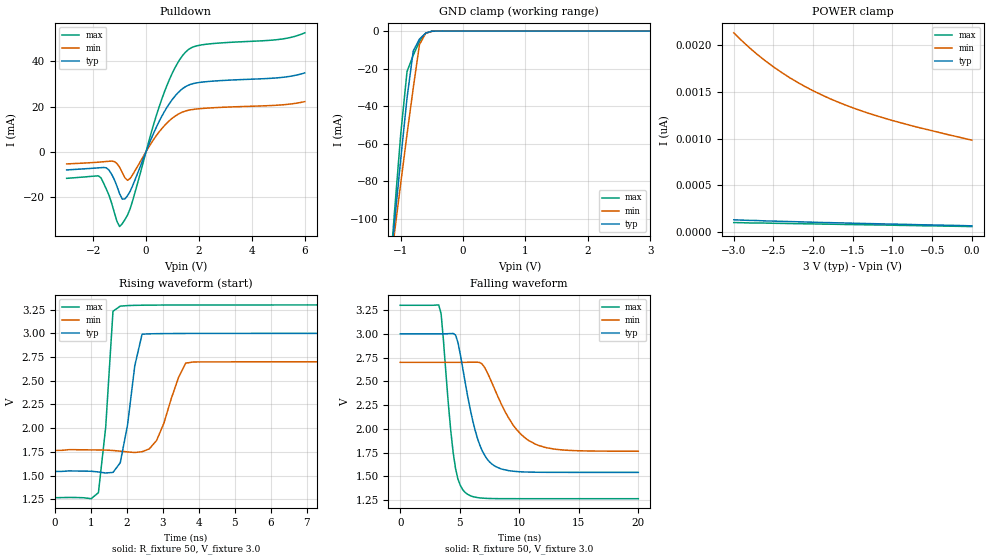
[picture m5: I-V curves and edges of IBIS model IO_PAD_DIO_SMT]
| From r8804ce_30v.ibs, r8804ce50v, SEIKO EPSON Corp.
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[Model]   IO_PAD_DIO_SMT
Model_type I/O_open_drain
Enable Active-High
Polarity Non-Inverting
Vinh=2.64
Vinl=0.54
Vref=3.3
Vmeas=1.50
Rref=5000
C_comp   2.5p   2.0p   3.0p
[Temperature Range] 25   105   -40
[Voltage Range]   3.0   2.7   3.3
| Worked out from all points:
|   slope of the pulldown table from 0 to 0.45 V, typ, clamps not added: 36.6 ohm
|   GND clamp passes 1 mA (typ) near -0.59 V on its own axis
|   falling waveform, R_fixture 50, V_fixture 3.0: 20-80 % time 1.52ns typ, 2.47ns min, 886ps max; typ from 3 V to 1.54 V
|   rising waveform, R_fixture 50, V_fixture 3.0: 20-80 % time 333ps typ, 498ps min, 245ps max; typ from 1.54 V to 3 V
[Pulldown]
-3V       -8.089mA   -5.43mA    -11.82mA
-1.7V     -7.088mA   -4.564mA   -11.64mA
-1.4V     -8.196mA   -4.255mA   -19.3mA
-1V       -18.62mA   -6.885mA   -33.2mA
-800mV    -20.97mA   -11.57mA   -30.13mA
-600mV    -17.54mA   -11.87mA   -25.25mA
600mV     15.77mA    10.27mA    23.45mA
1.1V      24.7mA     15.77mA    37.31mA
1.5V      28.87mA    18.05mA    44.2mA
2.1V      30.79mA    19.12mA    47.31mA
5V        32.75mA    20.62mA    49.7mA
6V        34.91mA    22.17mA    52.66mA
[GND Clamp]
-3V       -764.1mA   -630.2mA   -940.2mA
-1.2V     -136mA     -134.3mA   -139.6mA
-1.1V     -101.9mA   -107.4mA   -96.17mA
-1V       -68.05mA   -80.96mA   -54.69mA
-900mV    -35.72mA   -55.09mA   -21.63mA
-800mV    -10.59mA   -30.38mA   -12.89mA
-700mV    -4.3mA     -7.21mA    -5.615mA
-600mV    -1.094mA   -1.181mA   -1.208mA
-500mV    -109.6uA   -173.5uA   -67.33uA
-400mV    -6.015uA   -18.81uA   -1.378uA
3V        67.42pA    1.041nA    53.55pA
[POWER Clamp]
-3V       132.1pA    2.129nA    102.5pA
-2.8V     125.7pA    1.968nA    98.45pA
-2.7V     124.1pA    1.896nA    98.23pA
-2.5V     118.5pA    1.765nA    95.04pA
-2.3V     113.1pA    1.652nA    92.31pA
-2.2V     111.3pA    1.602nA    90.27pA
-2V       106.2pA    1.51nA     88.33pA
-1.8V     102pA      1.43nA     85.27pA
-1.4V     93.68pA    1.298nA    79.69pA
-1V       86.74pA    1.192nA    74.58pA
-700mV    80.26pA    1.124nA    70.03pA
0V        67.42pA    982.3pA    59.57pA
[Falling Waveform]
R_fixture=50
V_fixture=3.0
V_fixture_min=2.7
V_fixture_max=3.3
0s        3V         2.7V       3.3V
3.232ns   3V         2.7V       3.304V
3.434ns   3V         2.7V       3.212V
4.444ns   3.003V     2.7V       1.754V
5.455ns   2.49V      2.7V       1.331V
6.667ns   1.836V     2.699V     1.275V
8.081ns   1.6V       2.375V     1.267V
9.697ns   1.553V     2.005V     1.266V
11.52ns   1.544V     1.831V     1.266V
20ns      1.543V     1.765V     1.266V
[Rising Waveform]
R_fixture=50
V_fixture=3.0
V_fixture_min=2.7
V_fixture_max=3.3
0s        1.543V     1.765V     1.266V
1.212ns   1.538V     1.77V      1.319V
1.414ns   1.527V     1.769V     2.01V
1.616ns   1.533V     1.764V     3.233V
1.818ns   1.635V     1.757V     3.287V
2.424ns   2.991V     1.751V     3.297V
2.828ns   2.996V     1.871V     3.298V
3.434ns   2.998V     2.532V     3.299V
3.838ns   2.999V     2.698V     3.299V
20ns      3V         2.7V       3.3V
[Ramp]
R_load=50
dV/dt_r   8.743E-1/2.997E-10   5.608E-1/4.811E-10   1.220E+0/1.913E-10
dV/dt_f   8.743E-1/1.518E-9   5.607E-1/2.466E-9   1.220E+0/8.767E-10
|[End   IO_PAD_DIO_SMT
